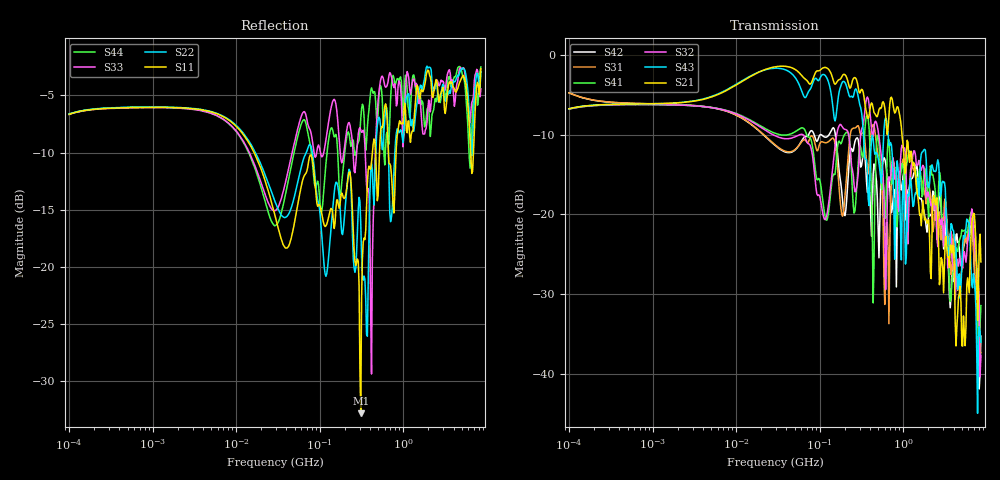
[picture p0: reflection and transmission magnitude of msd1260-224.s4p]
# MHz S MA R 50
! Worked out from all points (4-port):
!   498 points, 100 kHz to 8.5 GHz, reference 50 ohm
!   strongest paths, dB at 100 kHz, 1.698 MHz, 29.49 MHz, 500.7 MHz, 8.5 GHz:
!     S21: -6.7, -6.0, -1.5, -7.3, -25.9
!     S43: -6.7, -6.0, -1.6, -12.9, -36.0
!     S32: -6.8, -6.2, -10.1, -9.5, -37.7
!     S41: -6.8, -6.3, -9.8, -10.2, -31.4
!     S31: -4.7, -6.2, -11.3, -12.6, -37.3
!     S42: -4.7, -6.2, -11.4, -21.9, -35.3
!   lowest |S11| = -32.8 dB at 309.9 MHz (marker M1), VSWR 1.05, Z = 50.6 + j2.22 ohm
!   |S11| at or under -10 dB: 16.35 MHz to 427.3 MHz (410.9 MHz wide, 185 % of centre); 664.4 MHz to 821.5 MHz (157.1 MHz wide, 21.1 % of centre); 6.408 GHz to 6.931 GHz (522.5 MHz wide, 7.83 % of centre)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
0.1  0.4648 19.7  0.4611 20.6  0.5796 -16.3  0.4586 -160.3
     0.4611 20.6  0.4665 19.7  0.4594 -160.1  0.5794 -16.5
     0.5796 -16.3  0.4594 -160.1  0.464 19.8  0.4612 20.5
     0.4586 -160.3  0.5794 -16.5  0.4612 20.5  0.4662 19.8
309.9263  0.02288 73.3  0.5989 -64.1  0.316 -2.8  0.263 -3.8
          0.5989 -64.1  0.1553 -48.5  0.3206 30.8  0.1982 -17.8
          0.316 -2.8  0.3206 30.8  0.3969 -39.3  0.4673 -103.0
          0.263 -3.8  0.1982 -17.8  0.4673 -103.0  0.4441 0.8
2062.915  0.6889 -172.1  0.07307 109.0  0.1449 128.4  0.1702 175.8
          0.07307 109.0  0.7462 -172.4  0.127 132.1  0.09914 152.5
          0.1449 128.4  0.127 132.1  0.5108 -165.6  0.157 175.5
          0.1702 175.8  0.09914 152.5  0.157 175.5  0.4221 173.0
2905.739  0.593 96.6  0.05224 -78.0  0.09463 76.3  0.08918 36.6
          0.05224 -78.0  0.606 99.5  0.0943 63.6  0.09066 39.3
          0.09463 76.3  0.0943 63.6  0.6453 84.2  0.1587 24.4
          0.08918 36.6  0.09066 39.3  0.1587 24.4  0.5918 96.0
4484.409  0.6017 -64.6  0.02394 147.2  0.03342 -62.5  0.05875 -32.2
          0.02394 147.2  0.6899 -73.7  0.04802 -54.6  0.06681 -65.1
          0.03342 -62.5  0.04802 -54.6  0.647 -68.3  0.0338 175.5
          0.05875 -32.2  0.06681 -65.1  0.0338 175.5  0.7409 -83.1
6462.473  0.2961 170.4  0.07053 64.2  0.09076 102.6  0.1032 120.0
          0.07053 64.2  0.3322 153.4  0.09773 124.6  0.08981 92.5
          0.09076 102.6  0.09773 124.6  0.4822 70.9  0.04686 -97.6
          0.1032 120.0  0.08981 92.5  0.04686 -97.6  0.2989 78.4
8500  0.7366 -28.8  0.05043 -136.9  0.01358 -55.0  0.02679 -61.2
      0.05043 -136.9  0.7172 -38.8  0.01301 -23.7  0.01724 -69.9
      0.01358 -55.0  0.01301 -23.7  0.6005 -43.4  0.01583 133.6
      0.02679 -61.2  0.01724 -69.9  0.01583 133.6  0.7483 -44.2
